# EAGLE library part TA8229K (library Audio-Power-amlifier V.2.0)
TA8229K is an audio power IC with built-in two channels developed for portable radio cassette tape recorder with power ON/OFF switch. Thermal shut down protection circuit is built in.
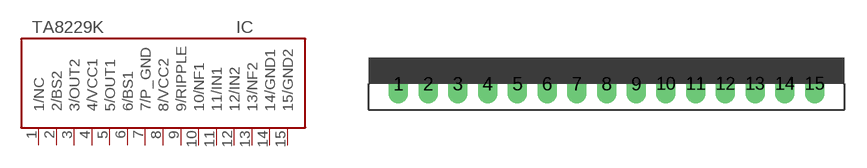
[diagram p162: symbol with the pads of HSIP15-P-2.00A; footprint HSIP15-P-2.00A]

Designator prefix IC

## TA8229K  [HSIP15-P-2.00A]
1  1/NC  nc
2  2/BS2  out
3  3/OUT2  out
4  4/VCC1  pwr
5  5/OUT1  out
6  6/BS1  out
7  7/P_GND  pwr
8  8/VCC2  pwr
9  9/RIPPLE
10  10/NF1  in
11  11/IN1  in
12  12/IN2  in
13  13/NF2  in
14  14/GND1  pwr
15  15/GND2  pwr

## Footprint HSIP15-P-2.00A (pad centres in mm)
drill 0.8 long: 1 -13.97,-1.27; 2 -11.97,-1.27; 3 -9.97,-1.27; 4 -7.97,-1.27; 5 -5.97,-1.27; 6 -3.97,-1.27; 7 -1.97,-1.27; 8 0.03,-1.27; 9 2.03,-1.27; 10 4.03,-1.27; 11 6.03,-1.27; 12 8.03,-1.27; 13 10.03,-1.27; 14 12.03,-1.27; 15 14.03,-1.27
